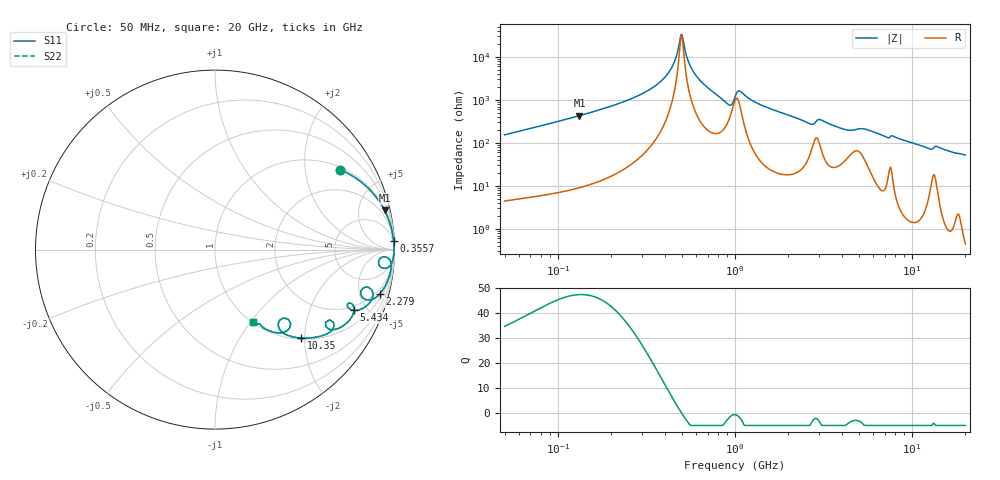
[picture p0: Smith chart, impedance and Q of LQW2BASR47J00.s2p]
!Murata Part Number: LQW2BASR47J00
!These Parameters are Measured in Series Mode Connection
!  o--[Z]--o
!Port1  Port2
!  o-------o
!Freq. Start=50[MHz] Stop=20[GHz], 401[Steps]
# Hz S RI R 50
!Freq.(Hz) S11(Real) S11(Imag) S21(Real) S21(Imag) S12(Real) S12(Imag) S22(Real) S22(Imag)
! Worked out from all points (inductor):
!   401 points, 50 MHz to 20 GHz, reference 50 ohm
!   read as one part in series: L = 483 nH near 51.52 MHz
!   highest Q = 47.4 at 132.4 MHz (marker M1), where L = 516 nH
!   self-resonance near 494.6 MHz
!   S11 on the Smith chart (normalised r, x): 50 MHz: 1.09, +3.08; 355.7 MHz: 3, +43; 2.279 GHz: 1.43, -7.26; 5.434 GHz: 1.75, -4.10; 10.35 GHz: 1.03, -1.92; 20 GHz: 1.01, -1.04
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5e7  0.6981 0.4449  0.3019 -0.4449  0.3019 -0.4449  0.6981 0.4449
1.323746e8  0.9444 0.2188  0.0556 -0.2188  0.0556 -0.2188  0.9444 0.2188
1.364002e8  0.9478 0.2122  0.0522 -0.2122  0.0522 -0.2122  0.9478 0.2122
3.557498e8  0.9953 0.0463  0.00473 -0.0463  0.00473 -0.0463  0.9953 0.0463
3.721004e8  0.9958 0.0401  0.00419 -0.0401  0.00419 -0.0401  0.9958 0.0401
4.387496e8  0.997 0.0175  0.00298 -0.0175  0.00298 -0.0175  0.997 0.0175
4.872511e8  0.9972 0.00326  0.00283 -0.00326  0.00283 -0.00326  0.9972 0.00326
5.020686e8  0.9971 -0.000859  0.00288 0.000859  0.00288 0.000859  0.9971 -0.000859
5.575697e8  0.9966 -0.0155  0.00344 0.0155  0.00344 0.0155  0.9966 -0.0155
6.380365e8  0.9947 -0.0355  0.00529 0.0355  0.00529 0.0355  0.9947 -0.0355
9.140482e8  0.9407 -0.1047  0.0593 0.1047  0.0593 0.1047  0.9407 -0.1047
1e9  0.9312 -0.042  0.0688 0.042  0.0688 0.042  0.9312 -0.042
1.061746e9  0.9686 -0.0512  0.0314 0.0512  0.0314 0.0512  0.9686 -0.0512
1.369645e9  0.9784 -0.1221  0.0216 0.1221  0.0216 0.1221  0.9784 -0.1221
2.279204e9  0.9172 -0.2478  0.0828 0.2478  0.0828 0.2478  0.9172 -0.2478
2.728004e9  0.8192 -0.2644  0.1808 0.2644  0.1808 0.2644  0.8192 -0.2644
2.98453e9  0.8678 -0.2182  0.1322 0.2182  0.1322 0.2182  0.8678 -0.2182
4.026975e9  0.7862 -0.3388  0.2138 0.3388  0.2138 0.3388  0.7862 -0.3388
5.433528e9  0.7742 -0.3362  0.2258 0.3362  0.2258 0.3362  0.7742 -0.3362
7.442007e9  0.6162 -0.4047  0.3838 0.4047  0.3838 0.4047  0.6162 -0.4047
1.034674e10  0.4801 -0.4924  0.5199 0.4924  0.5199 0.4924  0.4801 -0.4924
2e10  0.2141 -0.4059  0.7859 0.4059  0.7859 0.4059  0.2141 -0.4059
